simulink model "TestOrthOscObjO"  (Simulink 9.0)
settings: Solver=FixedStepDiscrete  StartTime=0.0  StopTime=10000  FixedStep=Tstep  RelTol=1e-3  EnableMultiTasking=on
InitFcn:
  | TestOrthOscObjO.TestOrthOscObjO_init();
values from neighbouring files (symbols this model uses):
  Tfq = 0.020    (= 0.02)    [TestOrthOscObjO_init.m]
  Tinit = 0.100    (= 0.1)    [TestOrthOscObjO_init.m]    (also in TestWaveMng_init.m)
  Tstep = 0.0005    [TestOrthOscObjO_init.m]    (also in TestWaveMng_init.m = 5e-05)
undefined symbols (not defined in the file or in its folder): TestOrthi
libraries: lib_OrthOsc x12, lib_AngleBlocks x9, lib_Inspc x6, lib_Conv x3, lib_T1Blocks_FB x2, simulink x1, lib_OObasics x1

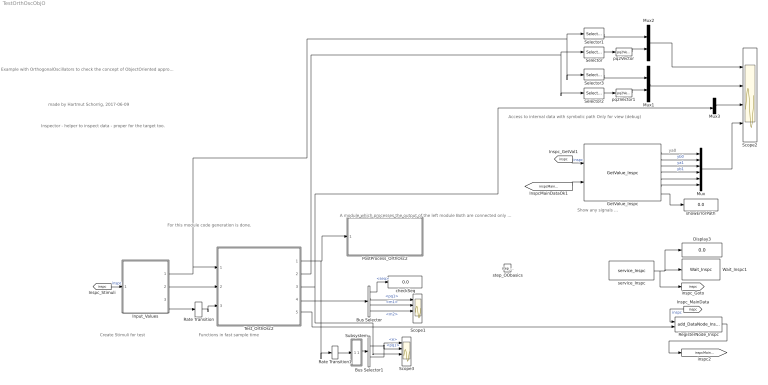
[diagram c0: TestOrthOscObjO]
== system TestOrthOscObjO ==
  note: ya0
  note: Inspector - helper to inspect data - proper for the target too.
  note: A module which processes the output of the left module Both are connected only via a handle in the Tinit time.
  note: Create Stimuli for test
  note: Show any signals ...
  note: made by Hartmut Schorrig, 2017-06-09
  note: Example with OrthogonalOscillators to check the concept of ObjectOriented approach in Simulink with handles to connect the Object-FB with the Operation-FB.
  note: Functions in fast sample time
  note: Access to internal data with symbolic path Only for view (debug)
  note: For this module code generation is done.
  Bus Selector : BusSelector  OutputSignals=seq,pq1,m1,m2
  Bus Selector1 : BusSelector  OutputSignals=e,pq1
  Display3 : Display
  GetValue_Inspc : lib_Inspc/GetValue_Inspc  Tstep=Tstep  path1='main_data.osc1[1].yab.re'  path2='main_data.osc1[1].yab.im'  path3='main_data.osc2[1].yab.re'  path4='main_data.osc2[1].yab.im'  path5='main_data.osc3[1].yab.re'  path6='main_data.osc3[1].yab.im'
  Input_Values : Subsystem
  Mux : Mux  Inputs=6
  Mux1 : Mux  Inputs=2
  Mux2 : Mux  Inputs=2
  Mux3 : Mux  Inputs=2
  PostProcess_OrthOsc2 : Subsystem  TreatAsAtomicUnit=on
  Rate Transition : RateTransition  Deterministic=off  OutPortSampleTime=Tfq
  Rate Transition1 : RateTransition  Deterministic=off  OutPortSampleTime=Tstep
  RegisterNode_Inspc : lib_Inspc/add_DataNode_Inspc  name1Refl='main'  name2Refl='_data'
  Scope1 : Scope  NumInputPorts=4
  Scope2 : Scope  NumInputPorts=4
  Scope3 : Scope  NumInputPorts=4
  Selector : Selector  IndexMode=Zero-based  InputPortWidth=2  IndexOptions=Index vector (dialog)  Indices=[0]  OutputSizes=1
  Selector1 : Selector  IndexMode=Zero-based  InputPortWidth=2  IndexOptions=Index vector (dialog)  Indices=[0]  OutputSizes=1
  Selector2 : Selector  IndexMode=Zero-based  InputPortWidth=2  IndexOptions=Index vector (dialog)  Indices=[1]  OutputSizes=1
  Selector3 : Selector  IndexMode=Zero-based  InputPortWidth=2  IndexOptions=Index vector (dialog)  Indices=[1]  OutputSizes=1
  Subsystem : Subsystem
  Test_OrthOsc2 : Subsystem  LoadFcn=TestOrthi.genBus();  TreatAsAtomicUnit=on
  Wait_Inspc1 : lib_Inspc/Wait_Inspc  Tstep=Tstep  cyclesStart=9999999  delay_ms=0
  checkSeq : Display
  pq2Vector : lib_Conv/pq2Vector  SystemSampleTime=-1
  pq2Vector1 : lib_Conv/pq2Vector  SystemSampleTime=-1
  service_Inspc : lib_Inspc/service_Inspc  Tstep=Tstep  IpPort='UDP:0.0.0.0:60094'
  showErrorPath : Display
  step_OObasics : lib_OObasics/step_OObasics
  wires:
  Mux2/1 -> Scope2/1
  Test_OrthOsc2/3(ypq) -> Mux3/2, Scope3/3
  Input_Values/3(Out3) -> Rate Transition/1
  Input_Values/1(Out1) -> Selector3/1, Selector1/1, Test_OrthOsc2/1(x)
  Input_Values/2(Out2) -> Test_OrthOsc2/2(wi)
  Test_OrthOsc2/2(ypq2) -> Selector2/1, Selector/1
  pq2Vector/1 -> Mux2/2
  Selector/1 -> pq2Vector/1
  Test_OrthOsc2/1(ya3) -> Rate Transition1/1, PostProcess_OrthOsc2/1(In1)
  Selector1/1 -> Mux2/1
  pq2Vector1/1 -> Mux1/2
  Selector2/1 -> pq2Vector1/1
  Selector3/1 -> Mux1/1
  Mux1/1 -> Scope2/2
  [inspc] -> RegisterNode_Inspc/1  "inspc"
  Test_OrthOsc2/5(data_inspc) -> RegisterNode_Inspc/2
  [inspc] -> GetValue_Inspc/1  "inspc"
  Mux/1 -> Scope2/4
  GetValue_Inspc/7 -> showErrorPath/1
  GetValue_Inspc/1 -> Mux/1
  GetValue_Inspc/2 -> Mux/2  "yb0"
  GetValue_Inspc/3 -> Mux/3  "ya1"
  GetValue_Inspc/4 -> Mux/4  "yb1"
  GetValue_Inspc/6 -> Mux/6
  GetValue_Inspc/5 -> Mux/5
  Mux3/1 -> Scope2/3
  RegisterNode_Inspc/1 -> [inspcMainDataOk]
  [inspc] -> Input_Values/1(In1)  "inspc"
  [inspcMainDataOk] -> GetValue_Inspc/2
  service_Inspc/1 -> [inspc], Display3/1, Wait_Inspc1/1
  Rate Transition/1 -> Test_OrthOsc2/3(fq)
  Bus Selector/2 -> Scope1/1  "<pq1>"
  Bus Selector/3 -> Scope1/2  "<m1>"
  Bus Selector/4 -> Scope1/3  "<m2>"
  Bus Selector/1 -> checkSeq/1  "<seq>"
  Test_OrthOsc2/4(ya1) -> Bus Selector/1
  Rate Transition1/1 -> Subsystem/1(In1)
  Subsystem/1(Out1) -> Bus Selector1/1
  Bus Selector1/1 -> Scope3/1  "<e>"
  Bus Selector1/2 -> Scope3/2  "<pq1>"

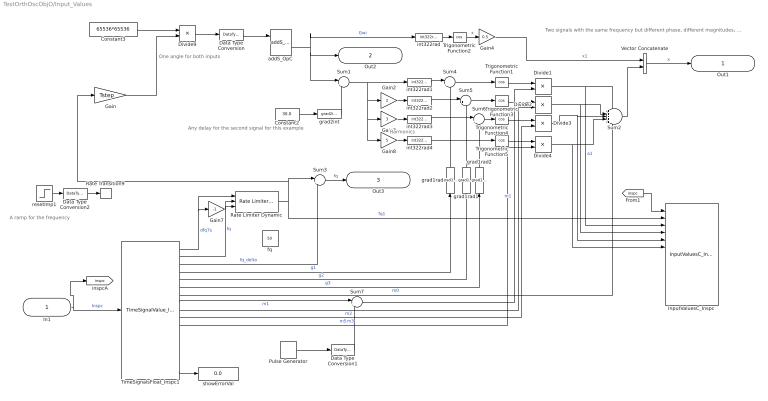
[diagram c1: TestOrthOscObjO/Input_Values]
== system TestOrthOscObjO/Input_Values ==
  note: A ramp for the frequency
  note: Two signals with the same frequency but different phase, different magnitudes, one signal has harmonics.
  note: Harmonics
  note: Any delay for the second signal for this example
  note: One angle for both inputs
  In1 : Inport  OutDataTypeStr=uint32
  Constant2 : Constant  Value=30.0  OutDataTypeStr=single
  Constant3 : Constant  Value=65536*65536  OutDataTypeStr=single
  Data Type Conversion : DataTypeConversion  OutDataTypeStr=int32
  Data Type Conversion1 : DataTypeConversion  OutDataTypeStr=single
  Data Type Conversion2 : DataTypeConversion  OutDataTypeStr=single
  Divide{1..4,9} (5 alike) : Product  Inputs=**
  Gain : Gain  Gain=Tstep
  Gain2 : Gain  Gain=2
  Gain3 : Gain  Gain=3
  Gain4 : Gain  Gain=0.5
  Gain7 : Gain  Gain=-1
  Gain8 : Gain  Gain=5
  InputValuesC_Inspc : lib_Inspc/InputValuesC_Inspc  Commented=on  nameRefl='testSignals'  n1='fq1'  n2='a1'  n3='a2'  n4='a3'  n5='a5'  n6='X6'  n7='X7'  n8='X8'  n9='X9'  n10='X10'  n11='X11'  n12='X12'
  Pulse Generator : DiscretePulseGenerator  PulseType=Time based  Amplitude=0.2  Period=1  PulseWidth=40
  Rate Limiter Dynamic : simulink/Discontinuities/Rate Limiter Dynamic
  Rate Transition9 : RateTransition  Integrity=off  Deterministic=off  OutPortSampleTime=Tfq
  Sum{1,3..7} (6 alike) : Sum  Inputs=|++
  Sum2 : Sum  Inputs=+++++
  TimeSignalsFloat_Inspc1 : lib_Inspc/TimeSignalValue_Inspc  Description=|  Tstep=Tstep  filepath=timeSignalFilepath  nameRefl='stimuli'  nrofStimuli=25  n1='dfq7s'  n2='fq'  n3='fq_delta'  n4='g1'  n5='g2'  n6='g3'  n7='m0'  n8='m1'  n9='m2'  n10='m3'  n11='m5'  n12=''  n13=''  n14=''  n15=''  n16=''
      | A combined stimuli and inspector function block.
      | Stimuli file path: file contains stimuli in form:
      |   %time:0: stimuli.namex = 5000.0, stimuli.namey = 50.0 -10; 
      | Name in reflection-tree: Name of this function block for stimuli and inspector access
      | name1..12: output type and name, base type is single always.
      | C2:namexy  A complex array of 2 elements
      | 6:namexy An array of 6 elements (max).
      | C:namexy  A 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
  Trigonometric Function{1..5} (5 alike) : Trigonometry  Operator=cos
  Vector Concatenate : Concatenate
  addS_OpC : lib_T1Blocks_FB/addS_OpC
  fq : Constant  Value=50  OutDataTypeStr=single
  grad1rad : lib_AngleBlocks/grad1rad
  grad1rad1 : lib_AngleBlocks/grad1rad
  grad1rad2 : lib_AngleBlocks/grad1rad
  grad2int : lib_AngleBlocks/grad2int
  int322rad{,1..4} (5 alike) : lib_AngleBlocks/int322rad
  resetImp1 : Step  Time=0.1  Before=0.995  After=1.2  SampleTime=Tfq
  showErrorVal : Display
  Out1 : Outport  OutDataTypeStr=single
  Out2 : Outport  Port=2  OutDataTypeStr=int32
  Out3 : Outport  Port=3  OutDataTypeStr=single
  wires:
  TimeSignalsFloat_Inspc1/3 -> Sum3/2  "fq_delta"
  In1/1 -> [inspc], TimeSignalsFloat_Inspc1/1  "Inspc"
  Constant3/1 -> Divide9/1
  int322rad/1 -> Trigonometric Function2/1
  Trigonometric Function2/1 -> Gain4/1  "x"
  Divide9/1 -> Data Type Conversion/1
  int322rad1/1 -> Sum4/1
  Trigonometric Function1/1 -> Divide1/1
  Constant2/1 -> grad2int/1
  Gain4/1 -> Vector Concatenate/1  "x1"
  Divide1/1 -> InputValuesC_Inspc/3, Sum2/1  "a1"
  Gain/1 -> Divide9/2
  Data Type Conversion/1 -> addS_OpC/1
  Data Type Conversion2/1 -> Rate Transition9/1
  Gain3/1 -> int322rad3/1
  Gain2/1 -> int322rad2/1
  int322rad2/1 -> Sum5/1
  int322rad3/1 -> Sum6/1
  Trigonometric Function3/1 -> Divide2/1
  Divide2/1 -> InputValuesC_Inspc/4, Sum2/2
  Trigonometric Function4/1 -> Divide3/1
  Divide3/1 -> InputValuesC_Inspc/5, Sum2/3
  Sum2/1 -> Vector Concatenate/2
  Rate Transition9/1 -> ?
  resetImp1/1 -> Data Type Conversion2/1
  grad2int/1 -> Sum1/2
  Vector Concatenate/1 -> Out1/1  "x"
  addS_OpC/2 -> int322rad/1, Sum1/1, Out2/1  "Gwi"
  [inspc] -> InputValuesC_Inspc/1
  Sum7/1 -> Divide1/2  "m1"
  TimeSignalsFloat_Inspc1/9 -> Divide2/2  "m2"
  TimeSignalsFloat_Inspc1/10 -> Divide3/2  "m3"
  Sum6/1 -> Trigonometric Function4/1
  TimeSignalsFloat_Inspc1/4 -> grad1rad/1  "g1"
  TimeSignalsFloat_Inspc1/5 -> grad1rad1/1  "g2"
  TimeSignalsFloat_Inspc1/6 -> grad1rad2/1  "g3"
  Sum5/1 -> Trigonometric Function3/1
  Sum4/1 -> Trigonometric Function1/1
  grad1rad/1 -> Sum4/2
  grad1rad1/1 -> Sum5/2
  grad1rad2/1 -> Sum6/2
  Rate Limiter Dynamic/1 -> Sum3/1, Gain/1, InputValuesC_Inspc/2  "fq1"
  TimeSignalsFloat_Inspc1/2 -> Rate Limiter Dynamic/2  "fq"
  Sum3/1 -> Out3/1  "fq"
  TimeSignalsFloat_Inspc1/1 -> Gain7/1, Rate Limiter Dynamic/1  "dfq7s"
  Gain7/1 -> Rate Limiter Dynamic/3
  Sum1/1 -> Gain8/1, Gain3/1, Gain2/1, int322rad1/1
  Gain8/1 -> int322rad4/1
  Trigonometric Function5/1 -> Divide4/1
  Divide4/1 -> InputValuesC_Inspc/6, Sum2/4
  int322rad4/1 -> Trigonometric Function5/1
  TimeSignalsFloat_Inspc1/11 -> Divide4/2  "m5"
  TimeSignalsFloat_Inspc1/7 -> Sum2/5  "m0"
  TimeSignalsFloat_Inspc1/17 -> showErrorVal/1
  Data Type Conversion1/1 -> Sum7/2
  TimeSignalsFloat_Inspc1/8 -> Sum7/1  "m1"
  Pulse Generator/1 -> Data Type Conversion1/1

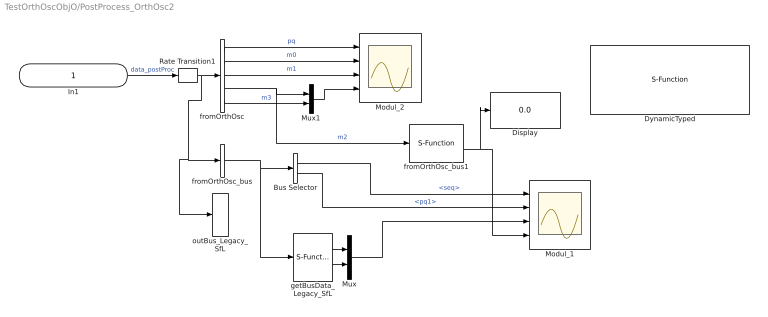
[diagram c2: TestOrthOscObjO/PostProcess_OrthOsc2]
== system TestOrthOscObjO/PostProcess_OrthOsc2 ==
  In1 : Inport  OutDataTypeStr=uint32
  Bus Selector : BusSelector  OutputSignals=seq,pq1
  Display : Display
  DynamicTyped : S-Function  Commented=on  FunctionName=getLocked_Output_Test_OrthOsc2_SfH  SFunctionDeploymentMode=off  EnableBusSupport=off
  Modul_1 : Scope  NumInputPorts=4
  Modul_2 : Scope  NumInputPorts=4
  Mux : Mux  Inputs=2
  Mux1 : Mux  Inputs=2
  Rate Transition1 : RateTransition  Integrity=off  OutPortSampleTime=Tfq
  fromOrthOsc : S-Function  FunctionName=getLocked_Output_Test_OrthOsc2_SfH  SFunctionDeploymentMode=off  EnableBusSupport=off
  fromOrthOsc_bus : S-Function  FunctionName=getSyncBus_Output_Test_OrthOsc2_SfH  SFunctionDeploymentMode=off  EnableBusSupport=off
  fromOrthOsc_bus1 : S-Function  FunctionName=step_Test_ArrayVoid_SmlkObjO_SfH  SFunctionDeploymentMode=off  EnableBusSupport=off
  getBusData_Legacy_SfL : S-Function  FunctionName=getBusData_Legacy_SfL  SFunctionDeploymentMode=off  EnableBusSupport=off
  outBus_Legacy_SfL : S-Function  FunctionName=outBus_Legacy_SfL  SFunctionDeploymentMode=off  EnableBusSupport=off
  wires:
  In1/1 -> Rate Transition1/1  "data_postProc"
  fromOrthOsc/2 -> Modul_2/2  "m0"
  fromOrthOsc/4 -> fromOrthOsc_bus1/1, Mux1/1  "m2"
  fromOrthOsc/5 -> Mux1/2  "m3"
  fromOrthOsc/1 -> Modul_2/1  "pq"
  Rate Transition1/1 -> outBus_Legacy_SfL/1, fromOrthOsc_bus/1, fromOrthOsc/1
  Mux1/1 -> Modul_2/4
  fromOrthOsc/3 -> Modul_2/3  "m1"
  fromOrthOsc_bus/1 -> getBusData_Legacy_SfL/1, Bus Selector/1
  Bus Selector/1 -> Modul_1/1  "<seq>"
  Bus Selector/2 -> Modul_1/2  "<pq1>"
  getBusData_Legacy_SfL/1 -> Mux/1
  getBusData_Legacy_SfL/2 -> Mux/2
  Mux/1 -> Modul_1/3
  fromOrthOsc_bus1/2 -> Display/1, Modul_1/4

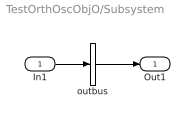
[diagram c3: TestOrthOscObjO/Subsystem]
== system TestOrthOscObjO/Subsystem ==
  In1 : Inport
  outbus : S-Function  FunctionName=getBus_Output_Test_OrthOsc2_SfH  SFunctionDeploymentMode=off  EnableBusSupport=off
  Out1 : Outport  OutDataTypeStr=Bus: Data_Output_Test_OrthOsc2
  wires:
  In1/1 -> outbus/1
  outbus/1 -> Out1/1

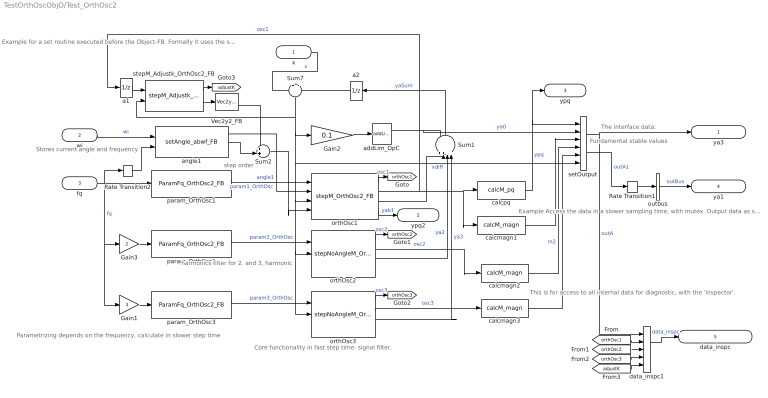
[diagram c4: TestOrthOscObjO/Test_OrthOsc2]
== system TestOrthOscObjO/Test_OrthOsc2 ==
  note: Example Access the data in a slower sampling time, with mutex. Output data as simulink bus
  note: The interface data:
  note: This is for access to all internal data for diagnostic, with the 'inspector'.
  note: Fundamental stable values
  note: harmonics filter for 2. and 3, harmonic
  note: Core functionality in fast step time: signal filter.
  note: Parametrizing depends on the frequency, calculate in slower step time
  note: Stores current angle and frequency
  note: Example for a set routine executed before the Object-FB. Formally it uses the stored thiz-reference from the last step time.
  note: step order
  x : Inport  OutDataTypeStr=single  PortDimensions=2  SampleTime=Tstep
  wi : Inport  Port=2  OutDataTypeStr=int32  SampleTime=Tstep
  fq : Inport  Port=3  OutDataTypeStr=single  SampleTime=Tfq
  Gain1 : Gain  Gain=3
  Gain2 : Gain  Gain=0.1
  Gain3 : Gain  Gain=2
  Rate Transition1 : RateTransition  Integrity=off  Deterministic=off  OutPortSampleTime=Tfq
  Rate Transition2 : RateTransition  Integrity=off  Deterministic=off  OutPortSampleTime=Tstep
  Sum1 : Sum  Inputs=++++|
  Sum2 : Sum  Inputs=++|
  Sum7 : Sum  Inputs=+|-
  Vec2y2_FB : lib_Conv/Vec2y2_FB  SystemSampleTime=-1
  a1 : UnitDelay  SampleTime=Tstep
  a2 : UnitDelay  SampleTime=Tstep
  addLim_OpC : lib_T1Blocks_FB/addLim_OpC  y0=0  lim=0.4
  angle1 : lib_OrthOsc/setAngle_abwf_FB  identObj=16  Tstep=Tstep
  calcmagn1 : lib_OrthOsc/calcM_magn
  calcmagn2 : lib_OrthOsc/calcM_magn
  calcmagn3 : lib_OrthOsc/calcM_magn
  calcpq : lib_OrthOsc/calcM_pq
  data_inspc1 : S-Function  FunctionName=set_Data_Test_OrthOsc2_SfH  Parameters=Tstep  SFunctionDeploymentMode=off  EnableBusSupport=off
  orthOsc1 : lib_OrthOsc/stepM_OrthOsc2_FB  ident=[21 22]  kA=2.0  kB=-2.0
  orthOsc2 : lib_OrthOsc/stepNoAngleM_OrthOsc2_FB  ident=[31 32]  kA=0.3  kB=-0.3
  orthOsc3 : lib_OrthOsc/stepNoAngleM_OrthOsc2_FB  ident=[41 42]  kA=0.3  kB=-0.3
  outbus : S-Function  FunctionName=getSyncBus_Output_Test_OrthOsc2_SfH  SFunctionDeploymentMode=off  EnableBusSupport=off
  param_OrthOsc1 : lib_OrthOsc/ParamFq_OrthOsc2_FB  identObj=17  Tstep=Tfq  TstepOrth=Tstep  m_nom=1
  param_OrthOsc2 : lib_OrthOsc/ParamFq_OrthOsc2_FB  identObj=18  Tstep=Tfq  TstepOrth=Tstep  m_nom=1
  param_OrthOsc3 : lib_OrthOsc/ParamFq_OrthOsc2_FB  identObj=19  Tstep=Tfq  TstepOrth=Tstep  m_nom=1
  setOutput : S-Function  FunctionName=set_Output_Test_OrthOsc2_SfH  Parameters=0  SFunctionDeploymentMode=off  EnableBusSupport=off
  stepM_Adjustk_OrthOsc2_FB : lib_OrthOsc/stepM_Adjustk_OrthOsc2_FB  ident=[21 22]  max_e=0.05  kHi=5  kNormal=2  Tdecay=0.1  Tstep=Tstep
  ya3 : Outport  OutDataTypeStr=uint32  SampleTime=Tinit
  ypq2 : Outport  Port=2  OutDataTypeStr=single  SampleTime=Tstep
  ypq : Outport  Port=3  OutDataTypeStr=single  SampleTime=Tstep
  ya1 : Outport  Port=4  OutDataTypeStr=Bus: Data_Output_Test_OrthOsc2
  data_inspc : Outport  Port=5  OutDataTypeStr=uint32  SampleTime=Tinit
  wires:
  fq/1 -> Gain3/1, Gain1/1, Rate Transition2/1, param_OrthOsc1/1  "fq"
  param_OrthOsc1/1 -> orthOsc1/1  "param1_OrthOsc"
  x/1 -> Sum7/1  "x"
  a2/1 -> Sum7/2
  wi/1 -> angle1/1  "wi"
  Sum1/1 -> a2/1  "yaSum"
  angle1/1 -> orthOsc1/2  "angle1"
  Gain3/1 -> param_OrthOsc2/1
  Gain1/1 -> param_OrthOsc3/1
  param_OrthOsc2/1 -> orthOsc2/1  "param2_OrthOsc"
  param_OrthOsc3/1 -> orthOsc3/1  "param3_OrthOsc"
  orthOsc2/3 -> Sum1/3  "ya2"
  orthOsc3/3 -> Sum1/4  "ya3"
  calcpq/1 -> ypq/1, setOutput/1  "ypq"
  Sum7/1 -> orthOsc3/2, orthOsc2/2, orthOsc1/3, setOutput/6, Gain2/1, stepM_Adjustk_OrthOsc2_FB/2  "xdiff"
  Rate Transition2/1 -> angle1/2
  orthOsc1/4 -> ypq2/1  "yab1"
  calcmagn2/1 -> setOutput/4  "m2"
  calcmagn3/1 -> setOutput/5
  setOutput/1 -> ya3/1, data_inspc1/1  "outA"
  data_inspc1/1 -> data_inspc/1  "data_inspc"
  calcmagn1/1 -> setOutput/3
  orthOsc1/2 -> a1/1, calcpq/1, calcmagn1/1  "osc1"
  orthOsc2/2 -> calcmagn2/1  "osc2"
  orthOsc3/2 -> calcmagn3/1  "osc3"
  orthOsc1/3 -> Sum1/2
  addLim_OpC/1 -> Sum1/1, setOutput/2  "ya0"
  Gain2/1 -> addLim_OpC/1
  angle1/2 -> Sum2/2
  outbus/1 -> ya1/1  "outBus"
  setOutput/2 -> Rate Transition1/1  "outA1"
  Rate Transition1/1 -> outbus/1
  a1/1 -> stepM_Adjustk_OrthOsc2_FB/1
  Sum2/1 -> orthOsc1/4
  stepM_Adjustk_OrthOsc2_FB/2 -> Vec2y2_FB/1
  Vec2y2_FB/2 -> Sum2/1
  orthOsc1/1 -> [orthOsc1]  "osc1"
  orthOsc2/1 -> [orthOsc2]  "osc2"
  orthOsc3/1 -> [orthOsc3]  "osc3"
  stepM_Adjustk_OrthOsc2_FB/1 -> [adjustK]
  [orthOsc1] -> data_inspc1/2
  [orthOsc2] -> data_inspc1/3
  [orthOsc3] -> data_inspc1/4
  [adjustK] -> data_inspc1/5
